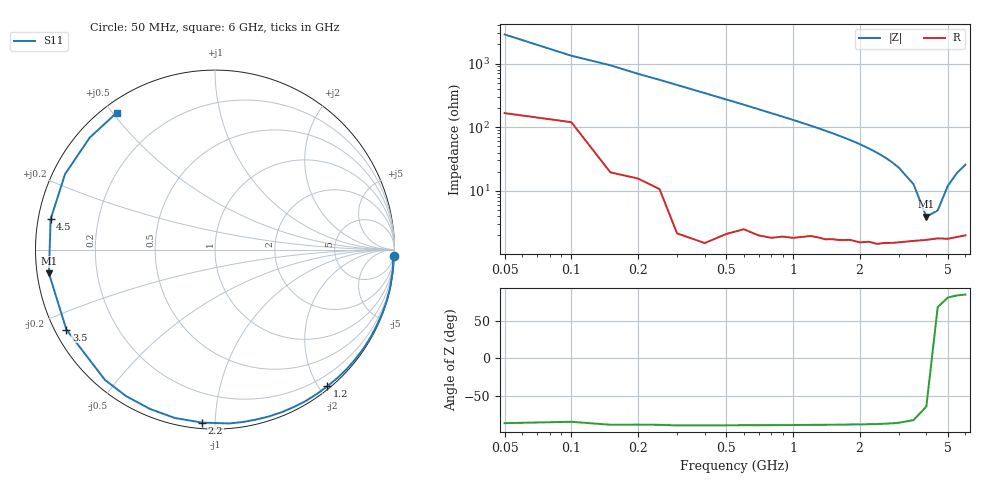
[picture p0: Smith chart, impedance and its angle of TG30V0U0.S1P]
! SIEMENS Discrete & RF Semiconductors
! BAT64
! Si Schottky Diode in SOT23
! VR = 30 V
! S-Parameters:  February  1997
# GHz  S  MA  R  50
!  f  S11
! GHz  MAG  ANG
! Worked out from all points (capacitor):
!   34 points, 50 MHz to 6 GHz, reference 50 ohm
!   read as one part to ground: C = 1.13 pF near 50 MHz
!   lowest |Z| = 3.92 ohm at 4 GHz (marker M1)
!   series resonance near 4.218 GHz, so ESL is about 1.3 nH
!   S11 on the Smith chart (normalised r, x): 50 MHz: 3, -57; 1.2 GHz: 0.04, -2.11; 2.2 GHz: 0.03, -0.93; 3.5 GHz: 0.03, -0.25; 4.5 GHz: 0.04, +0.09; 6 GHz: 0.04, +0.51
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0.05  0.998 -2.0
0.1  0.9932 -4.3
0.15  0.9978 -6.1
0.3  0.999 -12.4
0.4  0.9987 -16.6
0.5  0.9973 -20.8
0.6  0.9953 -25.0
0.7  0.9949 -29.3
0.8  0.9939 -33.6
1  0.9907 -42.0
1.2  0.9858 -50.6
1.3  0.9844 -54.8
1.4  0.9832 -59.2
1.6  0.9792 -67.8
1.7  0.9768 -72.2
1.9  0.973 -80.9
2  0.9719 -85.3
2.2  0.9665 -94.3
2.4  0.9646 -103.3
2.6  0.959 -112.2
2.8  0.9548 -121.3
3  0.9502 -130.2
3.5  0.9404 -151.7
4  0.9348 -171.9
4.5  0.9314 169.5
5  0.9354 153.3
5.5  0.9363 138.2
6  0.9386 125.7
